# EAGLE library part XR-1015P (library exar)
Seventh order switched capacitor FILTER
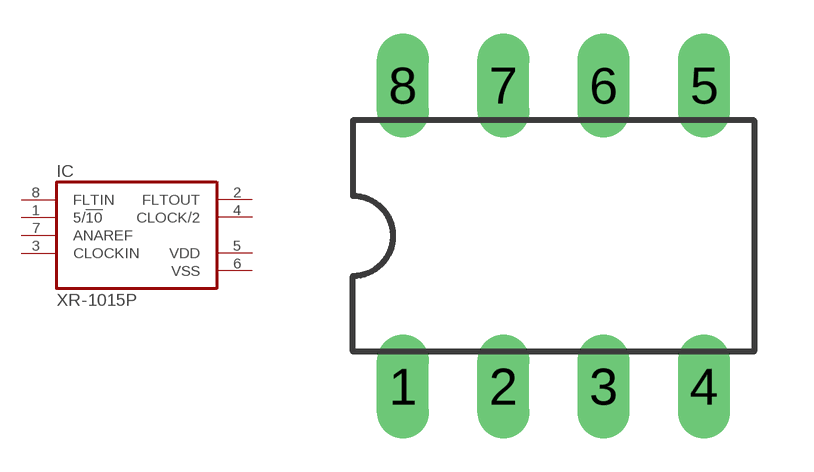
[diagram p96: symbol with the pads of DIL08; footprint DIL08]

Designator prefix IC

## XR-1015P (OC_FARNELL: unknown; OC_NEWARK: unknown)  [DIL08]
1  5/!10  in
2  FLTOUT  out
3  CLOCKIN  in
4  CLOCK/2  out
5  VDD  pwr
6  VSS  pwr
7  ANAREF  in
8  FLTIN  in

## Footprint DIL08 (pad centres in mm)
Dual In Line Package
drill 0.813 long: 1 -3.81,-3.81; 2 -1.27,-3.81; 3 1.27,-3.81; 4 3.81,-3.81; 5 3.81,3.81; 6 1.27,3.81; 7 -1.27,3.81; 8 -3.81,3.81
